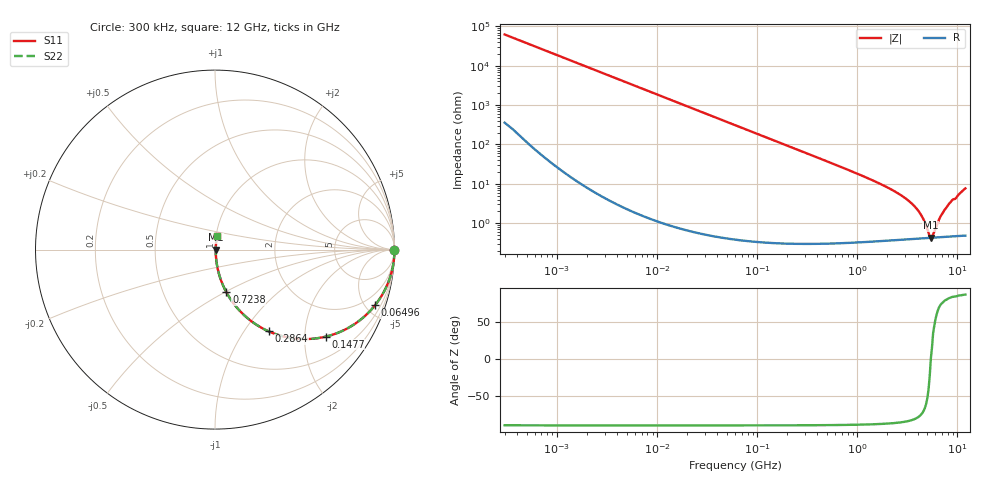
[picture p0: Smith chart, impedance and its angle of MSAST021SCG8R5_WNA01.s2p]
! MSAST021SCG8R5_WNA01  S-PARAMETER MODEL  ( General Type )
! Model Generated by TAIYO YUDEN Corporation (http://www.ty-top.com)
! Version 2.0
! TAIYO YUDEN Control No. 181101
! Copyright(c) 2015 TAIYO YUDEN CO.,LTD. All Rights Reserved.
! Product Description (link to TY-COMPAS)
! https://ds.yuden.co.jp/TYCOMPAS/or/detail?pn=MSAST021SCG8R5CWNA01&u=M
! Products Name : Multilayer Ceramic Capacitors
! Characteristics :
!  Capacitance : 8.5 pF , Rated Voltage : 25V , TCC : CG / C0G
!  Case Size : 0.25 x 0.125 / 0.0098 x 0.0049 [mm/inch] , Thickness : 0.125 / 0.0049 [mm/inch]
!  (Conditions: Temperature = 25 degC , DC Bias Current/Voltage = 0A / 0V)
! External Node Assignments :
!  1  o---| |---o  2
! GND o---------o GND
! Frequency Range : 0.3MHz  -  12000MHz  [ 401 STEP ]
# MHz S RI R 50
! Freq[MHz].  S11 Real  S11 Imag  S21 Real  S21 Imag  S12 Real  S12 Imag  S22 Real  S22 Imag
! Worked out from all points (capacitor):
!   401 points, 300 kHz to 12 GHz, reference 50 ohm
!   read as one part in series: C = 8.5 pF near 316.3 kHz
!   lowest |Z| = 427 mohm at 5.42 GHz (marker M1)
!   series resonance near 5.421 GHz, so ESL is about 100 pH
!   S11 on the Smith chart (normalised r, x): 300 kHz: open; 64.96 MHz: 1.01, -5.76; 147.7 MHz: 1.01, -2.53; 286.4 MHz: 1.01, -1.30; 723.8 MHz: 1.01, -0.51; 12 GHz: 1.01, +0.15
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0.3  1 -0.0016  1.18e-05 0.0016  1.18e-05 0.0016  1 -0.0016
1.769972  0.9999 -0.00945  9.79e-05 0.00945  9.79e-05 0.00945  0.9999 -0.00945
10.44266  0.9969 -0.0556  0.00313 0.0556  0.00313 0.0556  0.9969 -0.0556
26.39317  0.9804 -0.1382  0.0196 0.1382  0.0196 0.1382  0.9804 -0.1382
60  0.9066 -0.2904  0.0934 0.2904  0.0934 0.2904  0.9066 -0.2904
64.96309  0.8922 -0.3095  0.1078 0.3095  0.1078 0.3095  0.8922 -0.3095
96.65937  0.7891 -0.4071  0.2109 0.4071  0.2109 0.4071  0.7891 -0.4071
147.6816  0.6159 -0.4852  0.3841 0.4852  0.3841 0.4852  0.6159 -0.4852
286.3882  0.2991 -0.4556  0.7009 0.4556  0.7009 0.4556  0.2991 -0.4556
353.9943  0.2185 -0.4104  0.7815 0.4104  0.7815 0.4104  0.2185 -0.4104
723.8279  0.0632 -0.2373  0.9368 0.2373  0.9368 0.2373  0.0632 -0.2373
2088.533  0.00935 -0.0754  0.9907 0.0754  0.9907 0.0754  0.00935 -0.0754
3026.31  0.00564 -0.0422  0.9944 0.0422  0.9944 0.0422  0.00564 -0.0422
3841.137  0.0046 -0.0241  0.9954 0.0241  0.9954 0.0241  0.0046 -0.0241
4385.161  0.00432 -0.0147  0.9957 0.0147  0.9957 0.0147  0.00432 -0.0147
5140.631  0.00423 -0.00371  0.9958 0.00371  0.9958 0.00371  0.00423 -0.00371
5420.343  0.00426 -2.05e-06  0.9957 2.05e-06  0.9957 2.05e-06  0.00426 -2.05e-06
5715.274  0.0043 0.00296  0.9957 -0.00296  0.9957 -0.00296  0.0043 0.00296
6699.894  0.00458 0.0132  0.9954 -0.0132  0.9954 -0.0132  0.00458 0.0132
7854.144  0.00518 0.0256  0.9948 -0.0256  0.9948 -0.0256  0.00518 0.0256
8732.115  0.00593 0.0365  0.9941 -0.0365  0.9941 -0.0365  0.00593 0.0365
12000  0.0105 0.0752  0.9895 -0.0752  0.9895 -0.0752  0.0105 0.0752
